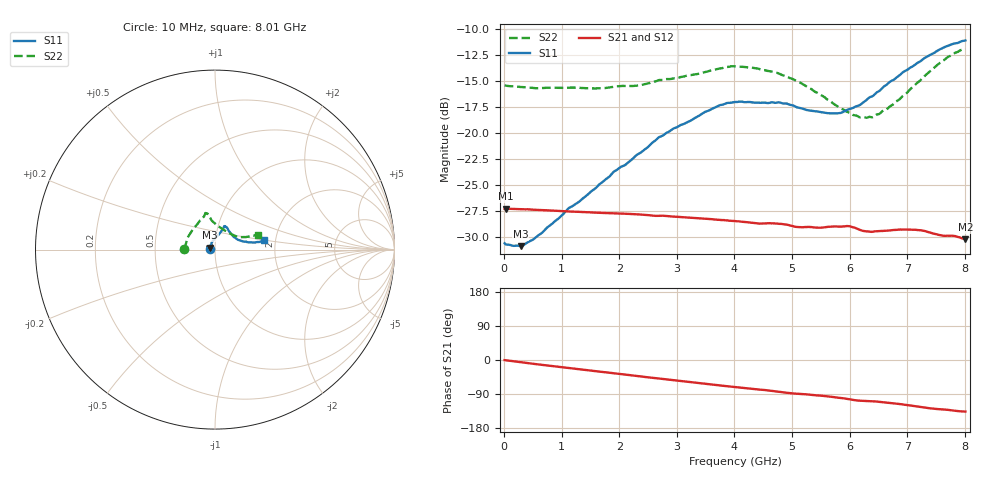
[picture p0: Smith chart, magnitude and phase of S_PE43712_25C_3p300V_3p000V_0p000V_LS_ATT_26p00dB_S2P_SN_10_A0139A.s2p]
! DEVICE ID: PE43712
! File Path: z:\PE43713\PE43713_CHAR_NOM_04292014\AMB\3p300\LS_ATT_26p00dB\PE43713_AMB_3p300V_3p000V_0p000V_LS_ATT_26p00dB_S2P_SN_10_A0139A.s2p
! Serial: 10
! Lot: A0139A
! Temp: 25C
! VDD: 3.300
! VSS: 0.000
! Control_Hi: 3.000
! Control_Lo: 0.000
! Attenuation Step: 26.00dB
! Port 1: RF1
! Port 2: RF2
! ThroughPath:1-2
! IDD: 0.00014524
! ISS: -6.48e-008
#  Hz  S  RI  R  50
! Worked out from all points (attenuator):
!   801 points, 10 MHz to 8.01 GHz, reference 50 ohm
!   highest |S21| = -27.26 dB at 30 MHz (marker M1); lowest = -30.2 dB at 8.01 GHz (marker M2)
!   lowest |S11| = -30.9 dB at 290 MHz (marker M3), VSWR 1.06, Z = 47.4 + j1.03 ohm
!   |S11| at or under -10 dB: start of sweep to end of sweep
!   |S22| runs from -18.5 to -11.9 dB; largest |S21 - S12| = 0.00016
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1e7  -0.0295 0.000792  0.0434 -0.000217  0.0434 -0.000194  -0.17 0.00119
3e7  -0.0291 0.00194  0.0434 -0.000494  0.0434 -0.000505  -0.1695 0.00295
2.9e8  -0.0265 0.0109  0.0429 -0.00436  0.0429 -0.00436  -0.166 0.0191
6.3e8  -0.0236 0.0227  0.0418 -0.00909  0.0418 -0.00908  -0.1601 0.0397
1.12e9  -0.0179 0.0397  0.0392 -0.0152  0.0392 -0.0152  -0.1507 0.069
1.35e9  -0.0133 0.0462  0.0378 -0.0179  0.0378 -0.0179  -0.1442 0.0808
2.28e9  0.0131 0.0765  0.0305 -0.0271  0.0304 -0.0271  -0.107 0.1312
2.68e9  0.0267 0.0915  0.0265 -0.03  0.0265 -0.03  -0.0873 0.1576
3.5e9  0.0458 0.1186  0.0177 -0.0345  0.0177 -0.0345  -0.0593 0.1883
3.74e9  0.0496 0.1271  0.015 -0.0353  0.015 -0.0353  -0.0556 0.1975
4.01e9  0.0534 0.131  0.012 -0.0359  0.012 -0.0358  -0.0532 0.2035
4.75e9  0.0636 0.1256  0.00419 -0.0365  0.00422 -0.0365  -0.035 0.1919
5.35e9  0.0803 0.0998  -0.00143 -0.0353  -0.00144 -0.0353  -0.0175 0.1613
5.82e9  0.1012 0.0734  -0.00609 -0.035  -0.00603 -0.0351  0.0159 0.132
5.99e9  0.113 0.0657  -0.00839 -0.0347  -0.00832 -0.0347  0.0318 0.1221
6.17e9  0.1241 0.0568  -0.0102 -0.0328  -0.0101 -0.0328  0.0502 0.1085
6.4e9  0.1425 0.0503  -0.0109 -0.0318  -0.0108 -0.0318  0.0759 0.0924
6.68e9  0.1698 0.0436  -0.0131 -0.0314  -0.0131 -0.0314  0.1085 0.0774
7.19e9  0.2156 0.0398  -0.0186 -0.0287  -0.0186 -0.0286  0.162 0.07
7.56e9  0.2493 0.0436  -0.0207 -0.0249  -0.0207 -0.0248  0.204 0.0754
7.81e9  0.2659 0.0481  -0.022 -0.0233  -0.022 -0.0233  0.2282 0.0816
8.01e9  0.275 0.0521  -0.0222 -0.0215  -0.0221 -0.0215  0.2398 0.0829
